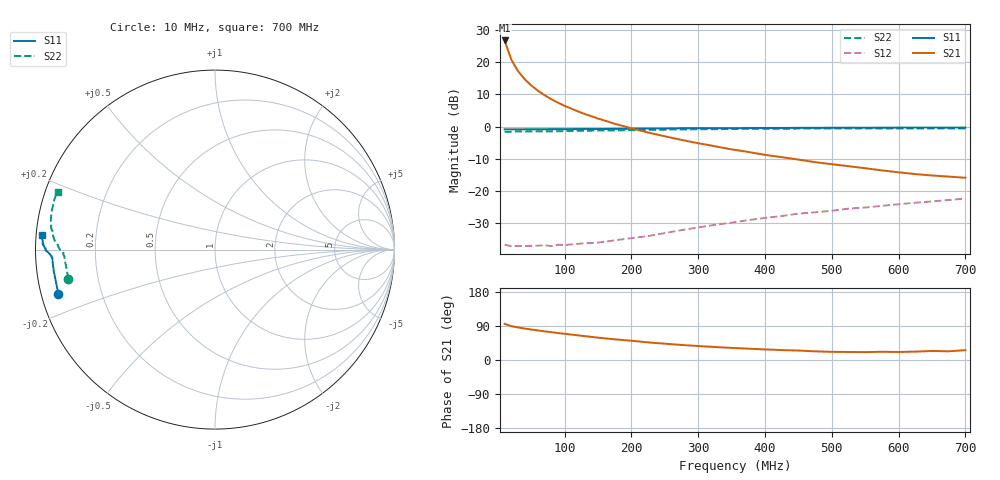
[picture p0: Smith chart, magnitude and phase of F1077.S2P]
! Date: Mon Aug 07 13:42:06 1995
# MHZ  S  MA  R  50.0000
!  POLYFET RF DEVICES
!  F1077
!  S PARAMETERS
!  VDS=28V, IDQ=1.20A
!FREQ  S11MAG S11ANG S21MAG S21ANG S12MAG S12ANG S22MAG S22ANG
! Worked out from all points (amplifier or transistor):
!   34 points, 10 MHz to 700 MHz, reference 50 ohm
!   highest |S21| = 26.7 dB at 10 MHz (marker M1)
!   |S21| within 3 dB of that: start of sweep to 15.06 MHz
!   unconditionally stable (mu >= 1): 148.7 MHz to 253.5 MHz
!   at 60 MHz: K = 0.51, MSG = 24.0 dB, |S12| = -36.9 dB
!   at 300 MHz: K = 0.88, MSG = 13.0 dB, |S12| = -31.2 dB
!   at 700 MHz: K = 0.76, MSG = 3.2 dB, |S12| = -22.3 dB
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10  0.907 -164.2  21.61 95.5  0.01483 9.7  0.8329 -168.7
20  0.9059 -171.9  10.91 89.3  0.01405 7.9  0.8355 -174.3
30  0.9067 -174.4  7.265 85.9  0.01412 9.8  0.8409 -176.2
40  0.9069 -175.8  5.439 83.0  0.0141 11.8  0.8386 -177.3
50  0.9076 -176.5  4.332 80.4  0.01421 13.4  0.8434 -177.8
60  0.9079 -177.1  3.593 77.9  0.01428 16.1  0.8458 -178.4
70  0.9099 -177.2  3.056 75.6  0.01454 17.1  0.8445 -178.6
80  0.9103 -177.6  2.653 73.4  0.01408 19.6  0.8464 -179.1
90  0.9127 -177.7  2.347 71.1  0.01478 23.4  0.8476 -179.2
100  0.9136 -177.8  2.093 69.1  0.01464 26.9  0.8522 -179.4
125  0.9178 -178.1  1.636 64.0  0.01545 31.7  0.8615 -179.9
150  0.918 -178.3  1.333 59.0  0.01597 39.4  0.8705 179.3
175  0.9229 -178.5  1.107 54.5  0.01729 45.2  0.8745 178.5
200  0.9286 -179.0  0.9402 50.8  0.01871 52.0  0.8813 177.9
225  0.932 -179.1  0.8094 46.4  0.02018 56.1  0.8908 177.1
250  0.9344 -179.4  0.7078 43.0  0.02242 59.8  0.8981 176.3
300  0.9438 -179.6  0.5524 36.9  0.02746 65.5  0.9107 174.3
375  0.9493 179.3  0.4048 29.9  0.03565 69.5  0.9234 171.8
475  0.9577 178.0  0.2811 22.9  0.04699 69.7  0.9327 167.9
500  0.9599 178.3  0.2618 21.5  0.04971 69.8  0.9339 166.8
600  0.9653 176.5  0.1958 21.2  0.06263 68.6  0.9383 163.5
700  0.9679 175.0  0.1612 26.0  0.0768 66.6  0.9325 160.0
